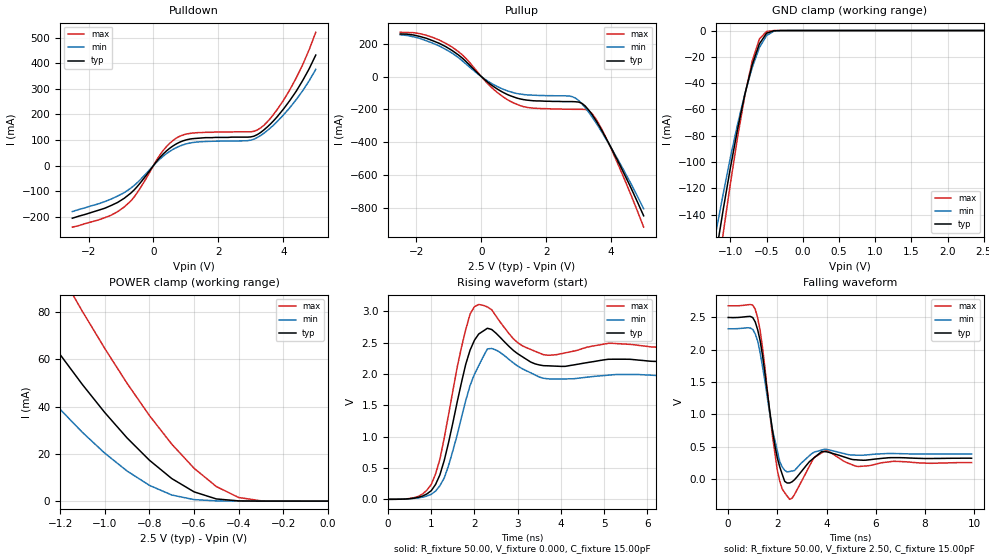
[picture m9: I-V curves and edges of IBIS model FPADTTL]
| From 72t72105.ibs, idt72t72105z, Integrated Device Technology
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|   Model FPADTTL
[Model]   FPADTTL
Model_type   3-state
Polarity   Non-Inverting
Enable   Active-High
Vmeas =  1.250V
C_comp   3.00pF   NA   NA
[Temperature Range]   25.00   85.00   -40.00
[Voltage Range]   2.50V   2.30V   2.70V
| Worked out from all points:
|   slope of the pulldown table from 0 to 0.375 V, typ, clamps not added: 6.94 ohm
|   slope of the pullup table from 0 to 0.375 V, typ, clamps not added: 6.23 ohm
|   GND clamp passes 1 mA (typ) near -0.45 V on its own axis
|   POWER clamp passes 1 mA (typ) near -0.50 V on its own axis
|   rising waveform, R_fixture 50.00, V_fixture 0.000, C_fixture 15.00pF: 20-80 % time 445ps typ, 472ps min, 423ps max; typ from 0 V to 2.2 V
|   falling waveform, R_fixture 50.00, V_fixture 2.50, C_fixture 15.00pF: 20-80 % time 466ps typ, 489ps min, 440ps max; typ from 2.5 V to 0.321 V
[Pulldown]
| voltage   I(typ)   I(min)   I(max)
-2.5V     -206mA     -180mA     -241mA
-1.5V     -167mA     -141mA     -204mA
-900mV    -128mA     -106mA     -162mA
-500mV    -82.28mA   -67.22mA   -106mA
300mV     45.13mA    36.58mA    59.01mA
800mV     90.82mA    75.57mA    114mA
1.4V      107mA      92.58mA    129mA
3V        112mA      99.27mA    132mA
3.4V      139mA      126mA      157mA
4.2V      254mA      226mA      296mA
4.6V      333mA      293mA      395mA
5V        432mA      376mA      521mA
[Pullup]
| voltage   I(typ)   I(min)   I(max)
-2.5V     260mA      255mA      270mA
-1.7V     234mA      219mA      252mA
-900mV    159mA      143mA      180mA
-500mV    97.12mA    81.41mA    116mA
200mV     -34.29mA   -27.66mA   -43.74mA
1V        -124mA     -98.21mA   -161mA
1.5V      -145mA     -112mA     -190mA
2.8V      -152mA     -122mA     -199mA
3.1V      -163mA     -166mA     -199mA
3.3V      -202mA     -215mA     -206mA
3.8V      -360mA     -367mA     -356mA
5V        -848mA     -805mA     -917mA
[GND_clamp]
| voltage   I(typ)   I(min)   I(max)
-2.5V     -663mA     -589mA     -765mA
-1.2V     -170mA     -153mA     -195mA
-1.1V     -136mA     -124mA     -154mA
-1V       -104mA     -96.2mA    -116mA
-900mV    -74.56mA   -70.77mA   -80.61mA
-800mV    -48.24mA   -47.88mA   -49.04mA
-700mV    -26.16mA   -28.23mA   -23.28mA
-600mV    -10.07mA   -12.98mA   -6.406mA
-500mV    -2.002mA   -3.724mA   -655uA
-400mV    -177uA     -538uA     -28.12uA
-300mV    -7.848uA   -44.31uA   -410nA
2.5V      25.16nA    97.83nA    24.47nA
[POWER_clamp]
| voltage   I(typ)   I(min)   I(max)
-2.5V     256mA      206mA      321mA
-1.6V     118mA      84.74mA    166mA
-1.4V     89.24mA    60.62mA    131mA
-1.3V     75.3mA     49.37mA    113mA
-1.2V     61.92mA    38.79mA    96.5mA
-1.1V     49.24mA    29.04mA    80.16mA
-800mV    17.3mA     6.679mA    36.2mA
-600mV    3.925mA    651uA      13.91mA
-500mV    924uA      114uA      6.162mA
-400mV    104uA      14.03uA    1.537mA
-300mV    6.378uA    1.193uA    142uA
0V        25.16nA    29.25nA    27nA
[Ramp]
| variable   typ   min   max
dV/dt_r   1.34/0.32n   1.20/0.34n   1.48/0.30n
dV/dt_f   1.32/0.35n   1.18/0.36n   1.48/0.35n
R_load = 50.00
[Rising Waveform]
R_fixture = 50.00
V_fixture = 0.000
C_fixture = 15.00pF
R_dut = 0.75
L_dut = 8.10nH
C_dut = 0.53pF
| time   V(typ)   V(min)   V(max)
0s        0V         0V         0V
1ns       138mV      80.99mV    238mV
1.3ns     619mV      340mV      977mV
1.8ns     2.159V     1.579V     2.713V
2.1ns     2.638V     2.134V     3.108V
2.4ns     2.709V     2.406V     3.024V
3ns       2.323V     2.126V     2.501V
3.6ns     2.132V     1.931V     2.307V
5.1ns     2.234V     1.981V     2.489V
9.9ns     2.202V     1.973V     2.436V
[Falling Waveform]
R_fixture = 50.00
V_fixture = 2.50
C_fixture = 15.00pF
R_dut = 0.75
L_dut = 8.10nH
C_dut = 0.53pF
| time   V(typ)   V(min)   V(max)
0s        2.5V       2.325V     2.681V
1.1ns     2.432V     2.247V     2.629V
1.4ns     1.907V     1.735V     2.024V
2ns       325mV      434mV      135mV
2.3ns     -37.27mV   134mV      -214mV
2.5ns     -61.66mV   116mV      -315mV
3.5ns     330mV      416mV      333mV
4ns       421mV      459mV      443mV
5.3ns     294mV      368mV      193mV
9.9ns     321mV      388mV      254mV
